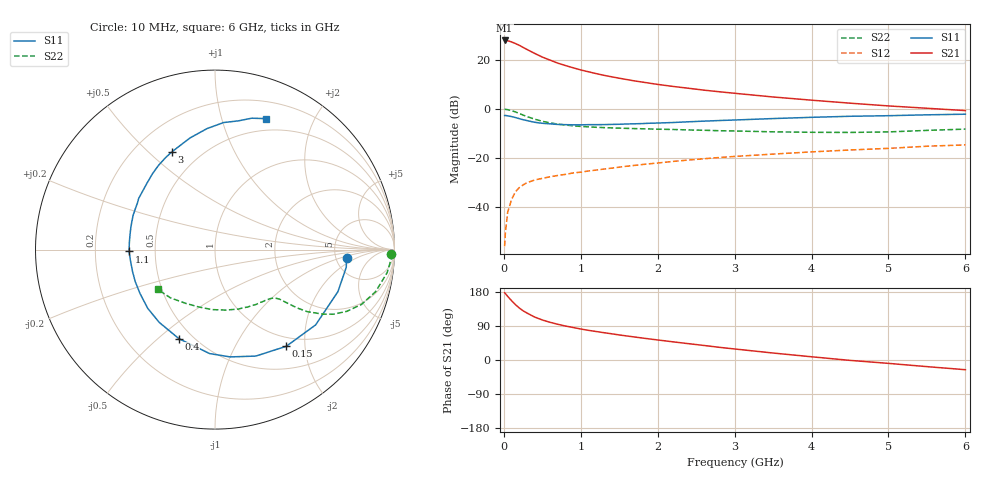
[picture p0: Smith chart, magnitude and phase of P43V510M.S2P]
! SIEMENS Small Signal Semiconductors
! BFP182
! Si NPN RF Bipolar Junction Transistor in SOT143
! VCE = 3.5 V  IC = 10 mA
! Common Emitter S-Parameters:  March  1996
# GHz  S  MA  R  50
!  f  S11  S21  S12  S22
! GHz  MAG  ANG  MAG  ANG  MAG  ANG  MAG  ANG
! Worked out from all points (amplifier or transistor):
!   36 points, 10 MHz to 6 GHz, reference 50 ohm
!   highest |S21| = 27.9 dB at 10 MHz (marker M1)
!   |S21| within 3 dB of that: start of sweep to 260.1 MHz
!   unconditionally stable (mu >= 1): 1.173 GHz to 5.375 GHz
!   at 250 MHz: K = 0.32, MSG = 28.0 dB, |S12| = -31.0 dB
!   at 1.4 GHz: K = 1.07, MAG = 17.0 dB, |S12| = -24.1 dB
!   at 6 GHz: K = 0.92, MSG = 7.0 dB, |S12| = -14.6 dB
!   lowest NFmin = 1.50 dB at 450 MHz
!   S11 on the Smith chart (normalised r, x): 10 MHz: 6.28, -1.26; 150 MHz: 0.84, -1.65; 400 MHz: 0.42, -0.59; 1.1 GHz: 0.35, -0.01; 3 GHz: 0.35, +0.59; 6 GHz: 0.37, +1.39
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0.01  0.7347 -3.6  24.9 177.5  0.0016 77.9  0.9816 -1.4
0.02  0.7379 -7.7  24.88 175.4  0.003 83.3  0.9829 -3.1
0.05  0.7238 -18.9  24.61 167.8  0.0079 82.9  0.9679 -7.6
0.1  0.7003 -36.8  23.22 156.6  0.0142 72.4  0.9249 -14.7
0.15  0.6692 -53.6  21.57 146.3  0.0205 66.1  0.8717 -20.5
0.2  0.6354 -69.0  19.88 137.3  0.0249 59.7  0.8108 -25.1
0.25  0.6039 -81.9  17.97 129.9  0.0283 56.1  0.7518 -28.6
0.3  0.5803 -92.9  16.34 124.0  0.0314 52.3  0.7005 -30.9
0.4  0.5353 -112.1  13.58 113.4  0.0357 47.9  0.62 -33.9
0.5  0.5109 -127.5  11.43 105.6  0.0385 45.4  0.561 -35.4
0.6  0.4975 -138.9  9.914 99.5  0.0415 44.6  0.5208 -36.1
0.7  0.4842 -149.6  8.601 94.3  0.0441 43.9  0.4918 -36.7
0.9  0.4754 -165.1  6.907 85.8  0.0497 44.0  0.4538 -37.5
1.1  0.4789 -178.8  5.725 78.3  0.0545 44.4  0.4316 -38.9
1.5  0.4879 162.1  4.231 66.1  0.0652 44.7  0.4071 -42.8
1.8  0.5039 149.1  3.536 58.0  0.0737 44.6  0.3951 -46.7
2.2  0.5297 135.7  2.878 47.9  0.0854 43.1  0.3821 -53.0
3  0.5957 113.7  2.088 29.1  0.1078 38.4  0.3558 -68.6
3.5  0.6375 102.6  1.755 18.4  0.1204 34.7  0.3422 -80.0
4.5  0.7096 86.1  1.313 -1.0  0.1459 27.5  0.3324 -106.2
5.5  0.76 74.4  1.034 -17.5  0.1741 20.2  0.3658 -132.6
6  0.7822 68.9  0.926 -25.6  0.1852 15.5  0.3886 -145.2
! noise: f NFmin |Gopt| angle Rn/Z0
0.45  1.5  0.26  43  0.28
0.9  1.6  0.24  87  0.22
1.8  2.1  0.2  170  0.2
